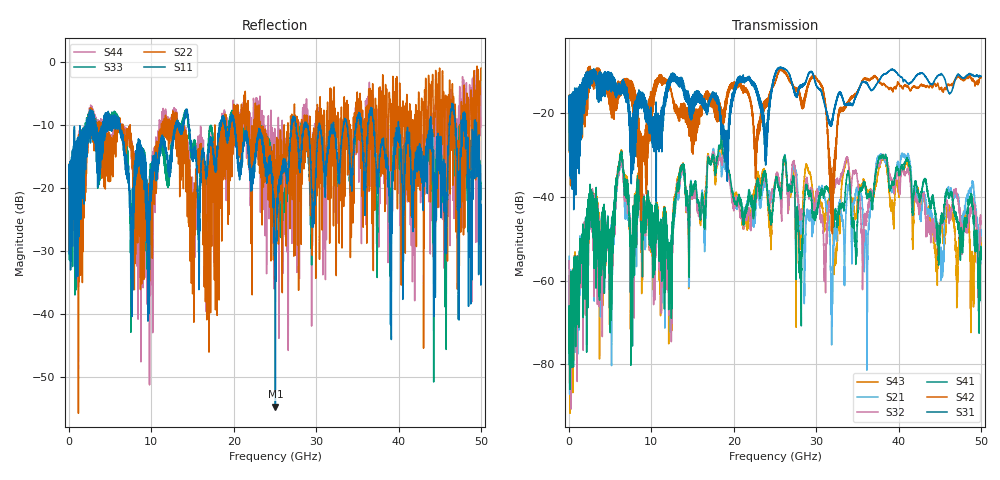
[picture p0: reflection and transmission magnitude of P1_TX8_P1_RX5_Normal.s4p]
!Keysight Technologies,N5225B,MY57041031,A.13.20.10
!Date: Friday, May 31, 2019 11:21:17
!Correction: S11(Full 4 Port(1,2,3,4))
!S12(Full 4 Port(1,2,3,4))
!S13(Full 4 Port(1,2,3,4))
!S14(Full 4 Port(1,2,3,4))
!S21(Full 4 Port(1,2,3,4))
!S22(Full 4 Port(1,2,3,4))
!S23(Full 4 Port(1,2,3,4))
!S24(Full 4 Port(1,2,3,4))
!S31(Full 4 Port(1,2,3,4))
!S32(Full 4 Port(1,2,3,4))
!S33(Full 4 Port(1,2,3,4))
!S34(Full 4 Port(1,2,3,4))
!S41(Full 4 Port(1,2,3,4))
!S42(Full 4 Port(1,2,3,4))
!S43(Full 4 Port(1,2,3,4))
!S44(Full 4 Port(1,2,3,4))
!S4P File: Measurements: <S11,S12,S13,S14>,
!<S21,S22,S23,S24>,
!<S31,S32,S33,S34>,
!<S41,S42,S43,S44>:
# Hz S  dB  R 50.0
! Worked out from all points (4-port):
!   5000 points, 10 MHz to 50 GHz, reference 50 ohm
!   strongest paths, dB at 10 MHz, 12.51 GHz, 25.01 GHz, 37.51 GHz, 50 GHz:
!     S31: -19.7, -10.8, -11.0, -12.7, -11.3
!     S42: -19.4, -15.6, -13.0, -12.4, -11.6
!     S41: -80.0, -52.3, -37.1, -31.8, -53.0
!     S32: -55.3, -58.4, -36.2, -32.5, -45.9
!     S21: -54.2, -51.9, -37.4, -30.7, -48.1
!     S43: -59.0, -57.0, -36.3, -34.3, -48.8
!   lowest |S11| = -54.7 dB at 25.05 GHz (marker M1), VSWR 1.00, Z = 49.8 + j0.0274 ohm
!   |S11| at or under -10 dB: 6.192 GHz to 12.89 GHz (6.695 GHz wide, 70.2 % of centre); 20.1 GHz to 26.99 GHz (6.893 GHz wide, 29.3 % of centre); 40 GHz to 43.77 GHz (3.766 GHz wide, 8.99 % of centre)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
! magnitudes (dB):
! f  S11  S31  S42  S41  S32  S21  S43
! 10 MHz  -19.4  -19.7  -19.4  -80.0  -55.3  -54.2  -59.0
! 6.26 GHz  -11.5  -15.8  -13.4  -30.3  -31.3  -31.3  -30.4
! 12.22 GHz  -17.6  -11.4  -13.5  -55.0  -62.3  -60.0  -55.7
! 25.05 GHz  -54.7  -10.5  -12.6  -36.5  -36.3  -36.8  -36.0
! 31.94 GHz  -10.5  -22.2  -36.2  -43.9  -37.5  -61.3  -44.9
! 37.79 GHz  -14.6  -11.9  -12.9  -30.4  -32.2  -30.5  -31.9
! 50 GHz  -22.6  -11.3  -11.6  -53.0  -45.9  -48.1  -48.8
